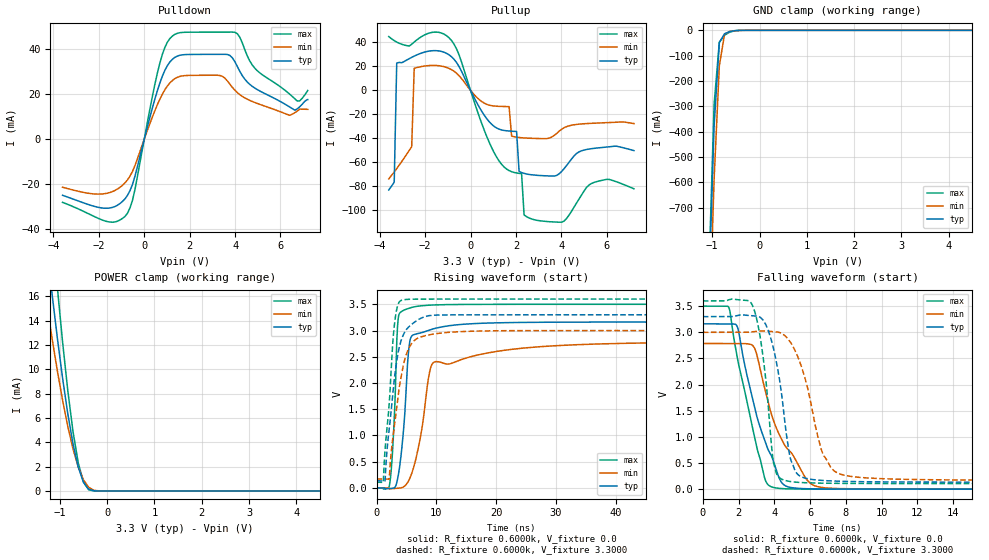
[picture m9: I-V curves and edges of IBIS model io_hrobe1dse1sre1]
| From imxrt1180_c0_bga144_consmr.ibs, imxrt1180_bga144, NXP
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[Model]  io_hrobe1dse1sre1
|   Model io_hrobe1dse1sre1
| This model was characterised for following simulation conditions:
| External (pad) voltage:
|   - Typ: 3.3V,   - Min: 3.0V,   - Max: 3.6V
| Library cells for typ/min/max conditions are connected as defined below:
|  PAD_IO - External Pad
|  ipp_do - Core Input
|  ipp_obe - Output Buffer Enable
|  ASRCN3V3[3] - NC
|  ASRCN3V3[4] - NC
|  ASRCP3V3[4] - NC
|  REFAPBIAS3V3 - gnde
|  REFBAMPL3V3 - vdd1v8
|  REFCAMPH3V3 - vdd1v8
|  REFDNBIAS3V3 - vdd1v8
|  REFH3V3 - REFH3V3
|  REFL3V3 - REFL3V3
|  gnde - gnde
|  ipp_dse - vdd
|  ipp_ina235_3v - NC
|  ipp_ina40_3v - NC
|  ipp_ina_mux - NC
|  ipp_ind - NC
|  ipp_ind_1p8v - NC
|  ipp_ind_3v - NC
|  ipp_sre - vdd
|  vdd - vdd
|  vdd1v8 - vdd1v8
|  vdda - vdde3v3
|  vdde3v3 - vdde3v3
| All other pins connected to ground
Model_type I/O
Polarity   Non-Inverting
Enable   Active-High
Vinl =   0.9900V
Vinh =   2.3100V
Vmeas =  1.6500V
Cref =   15.0000pF
Rref =   0.6000k
Vref =   0.0V
C_comp   4.0008pF   3.8189pF   4.1206pF
|C_comp_pullup   0.5642pF   0.7338pF   0.4701pF
|C_comp_pulldown   2.1153pF   2.2134pF   1.8990pF
[Model Spec]
| variable   typ   min   max
Vinh   2.3100V   NA   NA
Vinl   0.9900V   NA   NA
Vref   0.0V   0.0V   0.0V
Cref   15.0000pF   15.0000pF   15.0000pF
Rref   0.6000k   0.6000k   0.6000k
[Receiver Thresholds]
Vcross_high  =   0.0V
Vcross_low  =   0.0V
Vdiff_ac  =   0.0V
Vdiff_dc  =   0.0V
Tdiffslew_ac  =   0.0S
[Temperature Range]   25.0000   0.1250k   -40.0000
[Voltage Range]   3.3000V   3.0000V   3.6000V
[Pullup Reference]   3.3000V   3.0000V   3.6000V
[Pulldown Reference]   0.0V   0.0V   0.0V
[POWER Clamp Reference]   3.3000V   3.0000V   3.6000V
[GND Clamp Reference]   0.0V   0.0V   0.0V
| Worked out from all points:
|   slope of the pulldown table from 0 to 0.495 V, typ, clamps not added: 26.5 ohm
|   slope of the pullup table from 0 to 0.495 V, typ, clamps not added: 28.3 ohm
|   GND clamp passes 1 mA (typ) near -0.49 V on its own axis
|   POWER clamp passes 1 mA (typ) near -0.52 V on its own axis
|   rising waveform, R_fixture 0.6000k, V_fixture 0.0: 20-80 % time 1.18ns typ, 2.31ns min, 706ps max; typ from 0 V to 3.16 V
|   rising waveform, R_fixture 0.6000k, V_fixture 3.3000: 20-80 % time 1.98ns typ, 2.18ns min, 1.33ns max; typ from 0.133 V to 3.3 V
|   falling waveform, R_fixture 0.6000k, V_fixture 0.0: 20-80 % time 1.59ns typ, 1.94ns min, 1.32ns max; typ from 3.16 V to 0 V
|   falling waveform, R_fixture 0.6000k, V_fixture 3.3000: 20-80 % time 830ps typ, 1.23ns min, 635ps max; typ from 3.3 V to 0.133 V
[Pulldown]
|Voltage   I(typ)   I(min)   I(max)
-3.6V     -24.95mA   -21.38mA   -28.1mA
-1.73V    -30.7mA    -24.22mA   -36.35mA
-740mV    -24.98mA   -18.14mA   -32.92mA
-410mV    -16.5mA    -11.77mA   -22.36mA
690mV     24.99mA    17.78mA    33.89mA
1.02V     32.66mA    23.61mA    43.07mA
1.35V     36.31mA    26.85mA    46.53mA
3.33V     37.63mA    28.24mA    47.5mA
3.99V     34.37mA    21.72mA    47.42mA
5.09V     21.35mA    15.41mA    29.39mA
6.74V     13.43mA    12.45mA    16.89mA
7.2V      17.54mA    13.21mA    21.56mA
[Pullup]
|Voltage   I(typ)   I(min)   I(max)
-3.6V     -83.01mA   -73.82mA   44.86mA
-3.36V    -76.53mA   -68.01mA   41.48mA
-3.25V    22.81mA    -65.21mA   40.27mA
-2.59V    27.52mA    -46.92mA   38.49mA
-2.48V    28.55mA    18.36mA    40.31mA
-1.82V    32.75mA    20.69mA    47.77mA
-610mV    23.08mA    14.19mA    34.35mA
930mV     -28.25mA   -12.77mA   -47.7mA
2.03V     -34.28mA   -39.02mA   -68.87mA
2.25V     -68.52mA   -39.5mA    -69.46mA
2.36V     -69.2mA    -39.66mA   -103.9mA
7.2V      -50.23mA   -27.69mA   -82.07mA
[GND_clamp]
|Voltage   I(typ)   I(min)   I(max)
-3.6V     -19.67A    -19.55A    -20.65A
-1.07V    -1.013A    -1.224A    -956.3mA
-960mV    -377.1mA   -587.4mA   -291.7mA
-850mV    -48.21mA   -140.8mA   -46.94mA
-740mV    -13.57mA   -15.59mA   -19.22mA
-630mV    -5.137mA   -4.351mA   -7.235mA
-520mV    -1.276mA   -1.53mA    -1.554mA
-300mV    -4.403uA   -32.47uA   -997nA
7.2V      0A         0A         0A
[POWER_clamp]
|Voltage   I(typ)   I(min)   I(max)
-3.6V     102.5mA    81.21mA    131.1mA
-1.38V    23.81mA    18.18mA    31.78mA
-1.27V    19.88mA    15.26mA    26.56mA
-1.16V    16.12mA    12.48mA    21.52mA
-1.05V    12.56mA    9.868mA    16.71mA
-830mV    6.344mA    5.304mA    8.253mA
-720mV    3.878mA    3.458mA    4.888mA
-610mV    1.973mA    1.979mA    2.327mA
-500mV    725uA      918.2uA    733.4uA
-390mV    144.3uA    301.5uA    95.95uA
-170mV    198.2nA    4.056uA    20.28nA
7.2V      0A         0A         0A
[Ramp]
| variable   typ   min   max
dV/dt_r  1.8971/1.1809n   1.6671/2.3137n   2.1003/0.7064n
dV/dt_f  1.9001/0.8297n   1.6991/1.2276n   2.0958/0.6354n
R_load = 0.6000k
[Rising Waveform]
R_fixture= 0.6000k
V_fixture= 0.0
V_fixture_min= 0.0
V_fixture_max= 0.0
|time   V(typ)   V(min)   V(max)
0s        75.99nV    1.221uV    58.53nV
2.232ns   -13.67mV   -21.95mV   94.83mV
2.841ns   -4.567mV   -12.85mV   1.028V
3.569ns   195.1mV    -7.43mV    3.164V
4.533ns   1.122V     19.2mV     3.386V
5.684ns   2.848V     212.6mV    3.433V
7.39ns    2.954V     996.3mV    3.47V
8.893ns   3.012V     2.218V     3.484V
9.74ns    3.04V      2.403V     3.488V
60ns      3.162V     2.779V     3.5V
[Rising Waveform]
R_fixture= 0.6000k
V_fixture= 3.3000
V_fixture_min= 3.0000
V_fixture_max= 3.6000
|time   V(typ)   V(min)   V(max)
0s        133.2mV    168.1mV    107mV
1.136ns   132.6mV    168.1mV    106.8mV
1.43ns    137.9mV    167.8mV    729.3mV
2.11ns    1.113V     169mV      1.584V
2.973ns   2.08V      1.165V     3.09V
3.454ns   2.472V     1.604V     3.442V
4.012ns   2.771V     2.051V     3.568V
5.839ns   3.114V     2.747V     3.597V
10.04ns   3.295V     2.942V     3.599V
60ns      3.3V       3V         3.6V
[Falling Waveform]
R_fixture= 0.6000k
V_fixture= 0.0
V_fixture_min= 0.0
V_fixture_max= 0.0
|time   V(typ)   V(min)   V(max)
0s        3.162V     2.786V     3.5V
1.437ns   3.163V     2.786V     3.486V
1.905ns   3.126V     2.787V     2.562V
2.901ns   1.557V     2.693V     994.7mV
3.519ns   878.4mV    1.854V     157.3mV
4.074ns   406mV      1.205V     23.76mV
4.585ns   71.28mV    839mV      8.147mV
5.877ns   7.917mV    157.6mV    1.409mV
7.182ns   2.802mV    16.53mV    367.4uV
60ns      361.7nV    1.137uV    226.5nV
[Falling Waveform]
R_fixture= 0.6000k
V_fixture= 3.3000
V_fixture_min= 3.0000
V_fixture_max= 3.6000
|time   V(typ)   V(min)   V(max)
0s        3.3V       3V         3.6V
2.756ns   3.317V     3.01V      3.531V
3.353ns   3.241V     3.026V     2.584V
3.961ns   2.682V     3.013V     500.9mV
4.277ns   2.133V     2.998V     221.3mV
4.842ns   683.2mV    2.839V     149.2mV
5.675ns   216.3mV    2.175V     124mV
6.714ns   165.8mV    679mV      114.4mV
8.301ns   146mV      243.1mV    109.5mV
60ns      133.2mV    168.1mV    107mV
